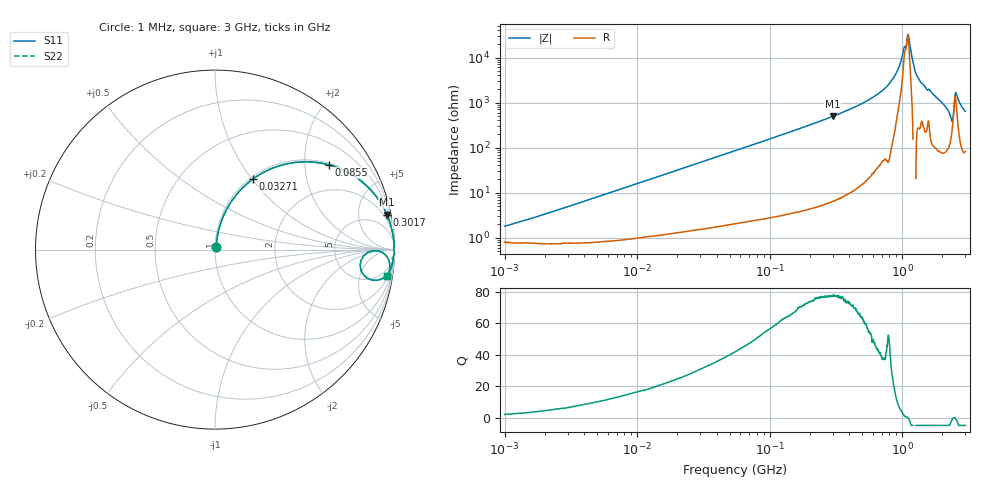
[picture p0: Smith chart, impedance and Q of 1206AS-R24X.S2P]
!s-Parameter Generated by FASTRON Sdn. Bhd.
!FASTRON P/N : 1206AS-R24X
!Keysight Technologies: E4991B_MY54100416_A.01.15
!Date created: Thu Nov 16 10:37:15 2023
!Version  : Rev00 Thu Nov 16 10:37:15 2023
!Data & Calibration Information:
!Freq	S11	S21	S12	S22
!PortZ  Port1:50+j0  Port2:50+j0
!When reading reference impedance value at option line is always used.
! Remarks : This data is being provided solely for informational purposes.
# Hz S dB R 50
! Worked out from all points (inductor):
!   1601 points, 1 MHz to 3 GHz, reference 50 ohm
!   read as one part in series: L = 255 nH near 1.427 MHz
!   highest Q = 77.4 at 298.7 MHz (marker M1), where L = 262 nH
!   self-resonance near 1.097 GHz
!   S11 on the Smith chart (normalised r, x): 1 MHz: 1.02, +0.03; 32.71 MHz: 1.03, +1.02; 85.5 MHz: 1.05, +2.64; 301.7 MHz: 1, +10; 3 GHz: 3, -13
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1000000  -35.00 62.9  -0.07 -0.9  -0.07 -0.9  -35.00 62.9
3804036  -24.33 79.5  -0.08 -3.5  -0.08 -3.5  -24.33 79.5
1.447069e7  -13.17 74.5  -0.31 -12.7  -0.31 -12.7  -13.17 74.5
3.271304e7  -6.98 61.7  -1.11 -26.6  -1.11 -26.6  -6.98 61.7
5.477226e7  -3.89 48.9  -2.45 -39.7  -2.45 -39.7  -3.89 48.9
8.550185e7  -2.05 36.7  -4.47 -52.2  -4.47 -52.2  -2.05 36.7
2.083556e8  -0.41 16.8  -10.78 -72.4  -10.78 -72.4  -0.41 16.8
2.987278e8  -0.20 11.5  -14.02 -77.8  -14.02 -77.8  -0.20 11.5
3.017325e8  -0.19 11.3  -14.12 -77.9  -14.12 -77.9  -0.19 11.3
5.555877e8  -0.05 5.0  -21.13 -83.9  -21.13 -83.9  -0.05 5.0
7.925923e8  -0.01 2.2  -28.13 -86.6  -28.13 -86.6  -0.01 2.2
9.255909e8  -0.02 1.1  -34.49 -82.7  -34.49 -82.7  -0.02 1.1
1.070143e9  -0.04 0.2  -45.09 -28.7  -45.09 -28.7  -0.04 0.2
1.108292e9  -0.03 -0.0  -50.26 14.3  -50.26 14.3  -0.03 -0.0
1.142072e9  -0.02 -0.3  -45.80 65.6  -45.80 65.6  -0.02 -0.3
1.262285e9  -0.00 -1.2  -33.33 89.1  -33.33 89.1  -0.00 -1.2
1.402151e9  -0.05 -2.1  -28.68 79.8  -28.68 79.8  -0.05 -2.1
2.061253e9  -0.13 -6.3  -19.19 78.9  -19.19 78.9  -0.13 -6.3
2.324278e9  -0.68 -10.6  -14.32 61.8  -14.32 61.8  -0.68 -10.6
2.383164e9  -1.50 -9.8  -13.04 39.9  -13.04 39.9  -1.50 -9.8
2.581816e9  -0.27 -3.4  -23.60 60.7  -23.60 60.7  -0.27 -3.4
3e9  -0.27 -8.7  -16.37 74.0  -16.37 74.0  -0.27 -8.7
